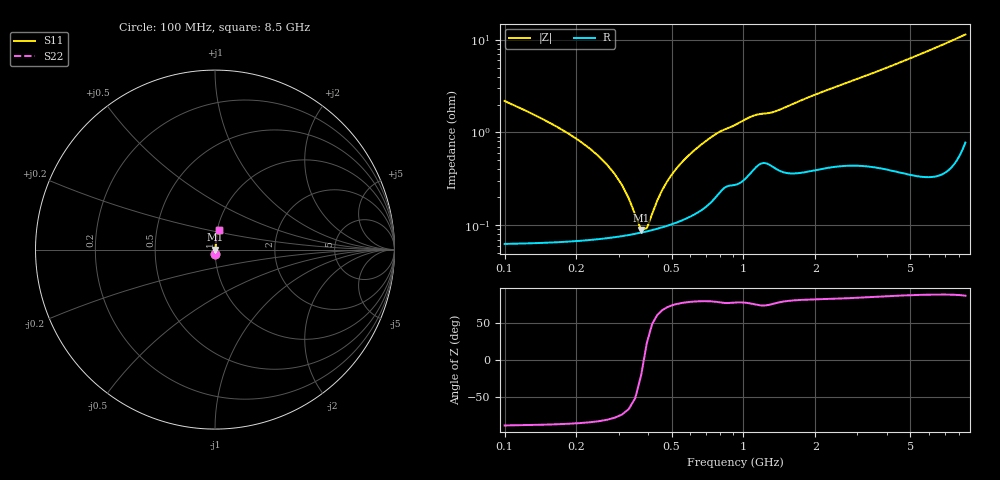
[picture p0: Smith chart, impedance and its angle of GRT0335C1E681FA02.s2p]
!Murata Part Number: GRT0335C1E681FA02
!These Parameters are Measured in Series Mode Connection
!Data Generated on Jun 19, 2026
!  o--ll--o
!Port1  Port2
!  o------o
!Operation Temp=25[degC], DC Bias Voltage=0[V]
!Freq. Start=100[MHz] Stop=9[GHz] 401[Steps]
# Hz S RI R 50
!Freq.(Hz) S11(Real) S11(Imag) S21(Real) S21(Imag) S12(Real) S12(Imag) S22(Real) S22(Imag)
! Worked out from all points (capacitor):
!   401 points, 100 MHz to 8.5 GHz, reference 50 ohm
!   read as one part in series: C = 680 pF near 142 MHz
!   lowest |Z| = 88.9 mohm at 373 MHz (marker M1)
!   series resonance near 382.9 MHz, so ESL is about 250 pH
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1e8  0.0011 -0.0218  0.9989 0.0218  0.9989 0.0218  0.0011 -0.0218
1.42e8  0.000844 -0.0142  0.9992 0.0142  0.9992 0.0142  0.000844 -0.0142
2.47e8  0.000736 -0.00553  0.9993 0.00553  0.9993 0.00553  0.000736 -0.00553
2.89e8  0.000753 -0.00348  0.9992 0.00348  0.9992 0.00348  0.000753 -0.00348
3.52e8  0.000806 -0.00103  0.9992 0.00103  0.9992 0.00103  0.000806 -0.00103
3.73e8  0.00083 -0.000316  0.9992 0.000316  0.9992 0.000316  0.00083 -0.000316
3.94e8  0.000856 0.000355  0.9991 -0.000355  0.9991 -0.000355  0.000856 0.000355
4.15e8  0.000885 0.000993  0.9991 -0.000993  0.9991 -0.000993  0.000885 0.000993
4.78e8  0.000988 0.00275  0.999 -0.00275  0.999 -0.00275  0.000988 0.00275
5.41e8  0.00112 0.00435  0.9989 -0.00435  0.9989 -0.00435  0.00112 0.00435
6.25e8  0.00135 0.00632  0.9987 -0.00632  0.9987 -0.00632  0.00135 0.00632
7.3e8  0.00182 0.00863  0.9982 -0.00863  0.9982 -0.00863  0.00182 0.00863
8.14e8  0.0025 0.0101  0.9975 -0.0101  0.9975 -0.0101  0.0025 0.0101
1.087e9  0.00398 0.0144  0.996 -0.0144  0.996 -0.0144  0.00398 0.0144
1.339e9  0.00443 0.016  0.9956 -0.016  0.9956 -0.016  0.00443 0.016
1.507e9  0.00398 0.0183  0.996 -0.0183  0.996 -0.0183  0.00398 0.0183
2.074e9  0.00465 0.026  0.9953 -0.026  0.9953 -0.026  0.00465 0.026
2.914e9  0.00567 0.0361  0.9943 -0.0361  0.9943 -0.0361  0.00567 0.0361
4.3e9  0.00664 0.0532  0.9934 -0.0532  0.9934 -0.0532  0.00664 0.0532
5.707e9  0.00847 0.0716  0.9915 -0.0716  0.9915 -0.0716  0.00847 0.0716
7.114e9  0.0121 0.0909  0.9879 -0.0909  0.9879 -0.0909  0.0121 0.0909
8.5e9  0.0202 0.1104  0.9798 -0.1104  0.9798 -0.1104  0.0202 0.1104
